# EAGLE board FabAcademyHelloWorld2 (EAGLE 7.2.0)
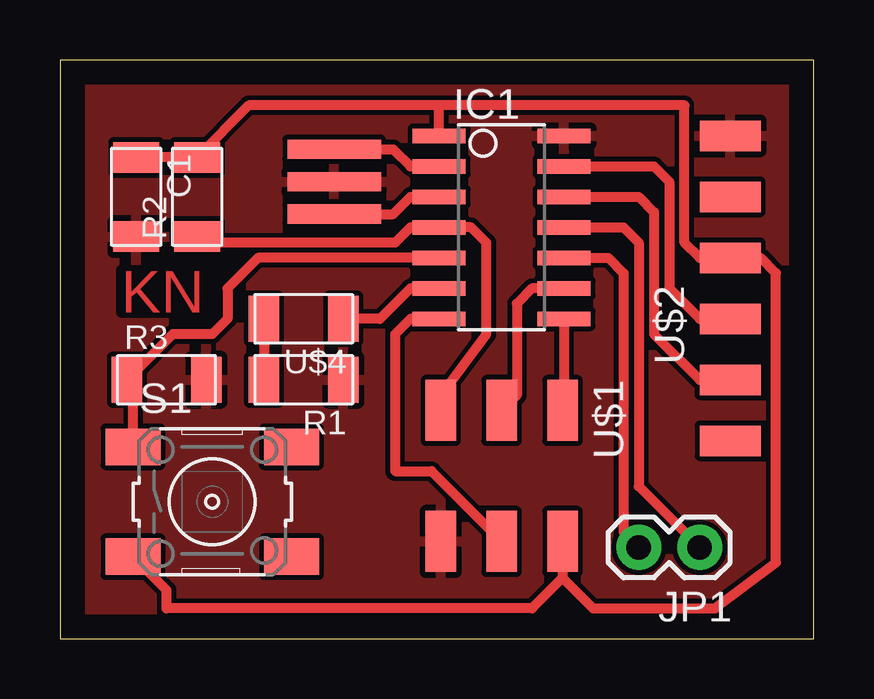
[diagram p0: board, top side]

Size 31.42 x 24.12 mm. Coordinates in mm from the lower left corner, seen from the top.
Outline: 0,0 31.42,0 31.42,24.12 0,24.12 0,0
Copper layers (1*16): Top 0.035mm / dielectric 1.5mm / Bottom 0.035mm
Design rules "default *": minimum track width 16mil, minimum drill 24mil, track to track 8mil, track to pad 8mil, pad to pad 8mil, via to via 8mil, smd to smd 8mil, copper to edge 40mil, drill to drill 8mil, minimum pad ring 10mil, minimum via ring 8mil, stop-mask expansion 4mil, vias tented up to drill 0mil, thermal gap 10mil

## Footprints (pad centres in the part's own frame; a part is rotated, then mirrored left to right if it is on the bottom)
C1206FAB = smd 1.27 x 1.905: 1 -1.651,0; 2 1.651,0
SOIC14 = smd 0.61 x 2.21: 1 -3.81,-2.603; 2 -2.54,-2.603; 3 -1.27,-2.603; 4 0,-2.603; 5 1.27,-2.603; 6 2.54,-2.603; 7 3.81,-2.603; 8 3.81,2.603; 9 2.54,2.603; 10 1.27,2.603; 11 0,2.603; 12 -1.27,2.603; 13 -2.54,2.603; 14 -3.81,2.603
1X02 = drill 1.016 pad 1.88: 1 0,0; 2 2.54,0
R1206FAB = smd 1.27 x 1.905: 1 -1.651,0; 2 1.651,0
6MM_SWITCH = smd 2.286 x 1.524: 1 -3.302,2.286; 2 3.302,2.286; 3 -3.302,-2.286; 4 3.302,-2.286
2X03SMD = smd 2.54 x 1.27: 1 -2.54,2.54; 2 2.92,2.54; 3 -2.54,0; 4 2.92,0; 5 -2.54,-2.54; 6 2.92,-2.54
1X06SMD = smd 2.54 x 1.27: 1 0,6.35; 2 0,3.81; 3 0,1.27; 4 0,-1.27; 5 0,-3.81; 6 0,-6.35
EFOBM = smd 0.8 x 3.9: 1 -1.35,0; 2 0,0; 3 1.35,0
LED1206FAB = smd 1.27 x 1.905: 1 -1.651,0; 2 1.651,0

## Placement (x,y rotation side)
C1  1uF  [C1206FAB]  3.18,18.41 270 top
IC1  ATTINY44-SSU  [SOIC14]  18.41,17.14 270 top
JP1  [1X02]  26.67,3.81 180 top
R1  499  [R1206FAB]  10.16,10.8 180 top
R2  10k  [R1206FAB]  5.71,18.41 90 top
R3  10k  [R1206FAB]  4.45,10.8 0 top
S1  [6MM_SWITCH]  6.35,5.71 0 top
U$1  AVRISPSMD  [2X03SMD]  18.41,6.98 270 top
U$2  FTDI-SMD-HEADER  [1X06SMD]  27.94,14.6 0 top
U$3  20MHz  [EFOBM]  11.43,19.05 270 top
U$4  LEDFAB1206  [LED1206FAB]  10.16,13.34 180 top

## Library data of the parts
C1 IC1 R1-R3 S1 U$1-U$4 = fablab
JP1 = SparkFun-Connectors

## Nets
BUTTON: IC1.5 R3.1 S1.1
CTS: U$2.2
GND: C1.2 IC1.14 R1.1 R3.2 U$1.6 U$2.1 U$3.2
LED: IC1.6 U$4.1
MISO: IC1.8 U$1.1
MOSI: IC1.7 U$1.4
N$1: R1.2 U$4.2
N$2: IC1.2 U$3.1
N$3: IC1.11 JP1.1
N$4: IC1.10 JP1.2
N$9: IC1.3 U$3.3
RESET: IC1.4 R2.1 U$1.5
RTS: U$2.6
RX: IC1.12 U$2.5
SCK: IC1.9 U$1.3
TX: IC1.13 U$2.4
VCC: C1.1 IC1.1 R2.2 S1.3 U$1.2 U$2.3

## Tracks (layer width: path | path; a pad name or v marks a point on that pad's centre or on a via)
BUTTON
  Top 0.406: S1.1 3.05,10.54 R3.1 4.7,12.7 6.35,12.7 6.98,13.34 6.98,14.6 8.26,15.88 IC1.5
GND
  pour Top: -1.27,25.4 32.38,25.4 32.38,-0.64 -1.27,-0.64
LED
  Top 0.406: IC1.6 14.61,14.6 13.34,13.34 U$4.1
MISO
  Top 0.406: IC1.8 21.02,9.59 U$1.1
MOSI
  Top 0.406: IC1.7 14.61,13.34 13.97,12.7 13.97,6.98 15.49,6.98 U$1.4
N$1
  Top 0.406: U$4.2 R1.2
N$2
  Top 0.406: U$3.1 13.89,20.4 14.61,19.69 IC1.2
N$3
  Top 0.406: IC1.11 23.49,17.14 24.13,16.51 24.13,6.35 JP1.1
N$4
  Top 0.406: IC1.10 22.86,15.88 23.49,15.24 23.49,4.45 JP1.2
N$9
  Top 0.406: U$3.3 13.89,17.7 14.61,18.41 IC1.3
RESET
  Top 0.406: R2.1 5.97,16.51 13.97,16.51 14.61,17.14 IC1.4 17.15,17.14 17.78,16.51 17.78,12.7 15.88,10.16 U$1.5
RX
  Top 0.406: IC1.12 24.13,18.41 24.77,17.78 24.77,12.7 26.67,10.8 U$2.5
SCK
  Top 0.406: IC1.9 19.69,14.6 19.05,13.97 19.05,10.16 U$1.3
TX
  Top 0.406: IC1.13 24.77,19.69 25.4,19.05 25.4,14.6 26.67,13.34 U$2.4
VCC
  Top 0.406: 20.95,2.54 19.69,1.27 4.45,1.27 4.45,2.03 S1.3 | 15.88,22.23 26.04,22.23 26.04,16.51 26.67,15.88 U$2.3 29.21,15.88 29.84,15.24 29.84,3.18 27.3,1.27 22.23,1.27 20.95,2.54 | 15.88,22.23 7.87,22.23 R2.2 C1.1 | IC1.1 15.81,22.16 15.88,22.23 | U$1.2 20.95,2.54

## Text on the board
Top: KN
